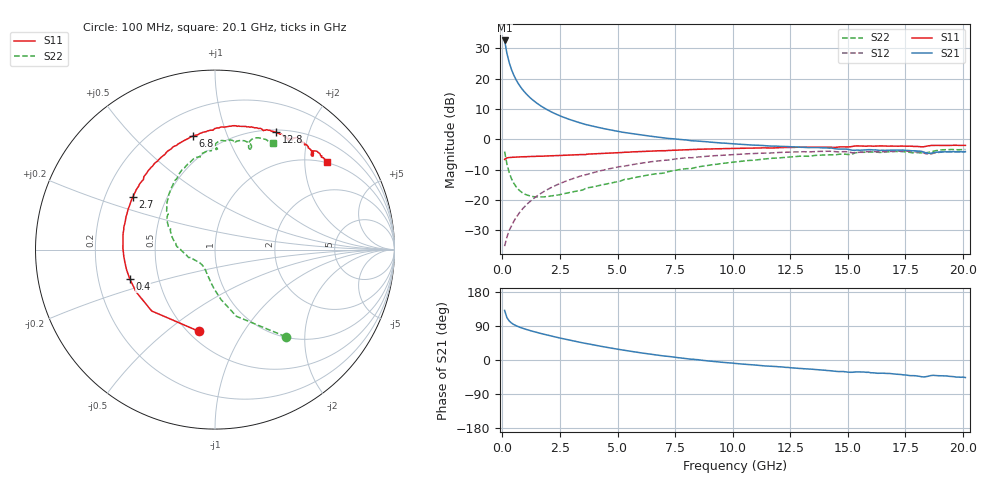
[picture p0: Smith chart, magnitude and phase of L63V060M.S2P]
!  Infineon Technologies AG
! BFR380L3 , PF131585-7, No.6, Th 09.10.01, soldered on pcb-board, measured with PP GSG850
!  Vce=3.0 V,  Ic=60.0 mA
! Common Emitter S-Parameters:  15. November 2001
#  GHz  S  MA  R  50
! f  S11  S21  S12  S22
! GHz  Mag  Ang  Mag  Ang  Mag  Ang  Mag  Ang
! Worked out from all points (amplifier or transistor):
!   201 points, 100 MHz to 20.1 GHz, reference 50 ohm
!   highest |S21| = 32.6 dB at 100 MHz (marker M1)
!   |S21| within 3 dB of that: start of sweep to 170.5 MHz
!   unconditionally stable (mu >= 1): 828.4 MHz to 4.117 GHz; 18.42 GHz to 18.52 GHz
!   at 3.4 GHz: K = 1.02, MAG = 8.0 dB, |S12| = -12.2 dB
!   at 10.1 GHz: K = 0.96, MSG = 1.7 dB, |S12| = -5.0 dB
!   at 20.1 GHz: K = 0.99, MSG = 0.0 dB, |S12| = -4.1 dB
!   S11 on the Smith chart (normalised r, x): 100 MHz: 0.56, -0.66; 400 MHz: 0.34, -0.15; 2.7 GHz: 0.32, +0.27; 6.8 GHz: 0.35, +0.76; 12.8 GHz: 0.53, +1.52; 20.1 GHz: 0.98, +2.57
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0.1  0.4645 -100.9  42.8 130.9  0.01713 57.3  0.6245 -50.9
0.2  0.4913 -135.9  26.23 111.7  0.02417 58.7  0.3903 -72.2
0.3  0.4988 -151.8  18.42 102.9  0.03118 61.3  0.281 -83.0
0.4  0.5022 -161.0  14.12 97.5  0.03728 63.9  0.2223 -90.7
0.5  0.5051 -166.9  11.4 93.5  0.0442 66.1  0.1869 -96.7
0.6  0.507 -171.7  9.56 90.5  0.05103 67.5  0.1638 -101.7
0.7  0.5093 -175.3  8.243 87.8  0.05793 68.4  0.148 -106.2
0.8  0.5111 -178.5  7.236 85.5  0.06508 69.2  0.1368 -110.2
0.9  0.5133 178.9  6.452 83.4  0.07229 69.6  0.1282 -113.7
1.1  0.5157 174.0  5.315 79.6  0.08653 69.8  0.119 -120.2
1.4  0.52 167.9  4.208 74.4  0.1079 69.3  0.1121 -128.2
1.7  0.5242 162.5  3.493 69.6  0.1293 68.2  0.1115 -135.0
2.1  0.5318 156.1  2.864 63.7  0.1577 66.2  0.1154 -142.4
2.7  0.5441 147.2  2.274 55.4  0.1991 62.7  0.1266 -152.6
3.5  0.5584 136.3  1.804 45.1  0.2532 57.2  0.1456 -162.5
5.1  0.5989 117.8  1.333 27.4  0.3526 45.6  0.2024 176.6
6.8  0.6449 100.8  1.077 12.2  0.4408 33.6  0.2723 155.9
10.1  0.7056 76.6  0.8349 -9.0  0.5606 11.6  0.4212 125.4
12.8  0.7385 62.5  0.7454 -21.8  0.6189 -5.3  0.522 102.8
13.5  0.7396 59.4  0.7294 -24.7  0.6242 -9.3  0.5346 98.4
16.8  0.7706 47.1  0.6624 -35.5  0.6289 -25.2  0.622 77.5
20.1  0.7925 38.0  0.6241 -46.2  0.6215 -38.9  0.677 61.3
